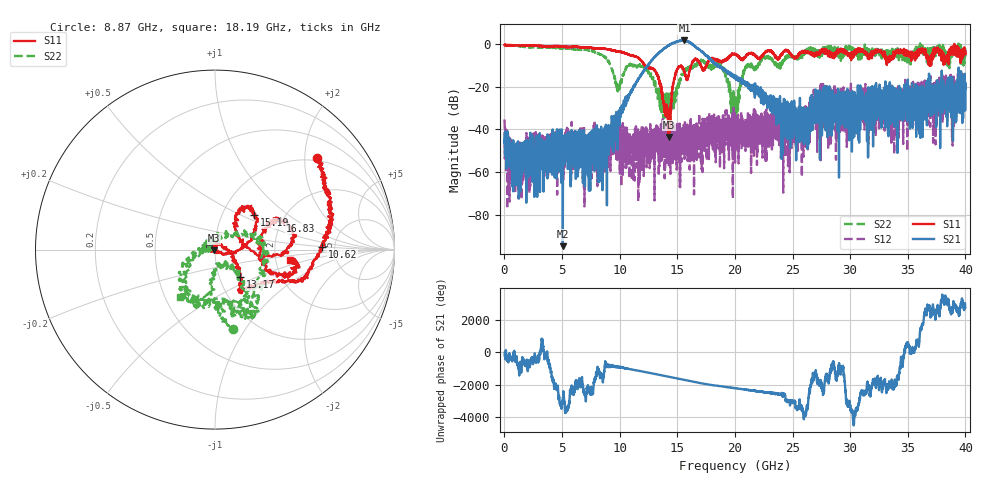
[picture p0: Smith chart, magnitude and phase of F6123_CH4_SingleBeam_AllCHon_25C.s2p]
!Keysight Technologies,N5245B,MY55451909,A.17.20.08
!Date: Tuesday, November 21, 2023 17:11:18
!Correction: S11(C  2-Port  )
!S21(C  2-Port  )
!S12(C  2-Port  )
!S22(C  2-Port  )
!S2P File: Measurements: S11, S21, S12, S22:
# Hz S  RI  R 50
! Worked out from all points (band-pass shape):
!   4000 points, 10 MHz to 40 GHz, reference 50 ohm
!   highest |S21| = 1.73 dB at 15.62 GHz (marker M1); lowest = -94.9 dB at 5.06 GHz (marker M2)
!   |S21| within 3 dB of the highest: 14.06 GHz to 16.57 GHz (2.514 GHz wide, 16.4 % of centre); 16.57504 GHz to 16.59008 GHz (15.04 MHz wide, 0.0907 % of centre)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
!   lowest |S11| = -43.5 dB at 14.26 GHz (marker M3), VSWR 1.01, Z = 49.5 - j0.431 ohm
!   |S11| at or under -10 dB: 12.21 GHz to 15.33 GHz (3.119 GHz wide, 22.7 % of centre); 15.33 GHz to 16.2 GHz (865.6 MHz wide, 5.49 % of centre); 17.04 GHz to 17.53 GHz (481.7 MHz wide, 2.79 % of centre)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
!   |S22| runs from -48.0 to 0.4 dB; largest |S21 - S12| = 1.2
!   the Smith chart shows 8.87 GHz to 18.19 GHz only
!   S11 on the Smith chart (normalised r, x): 8.87 GHz: 0.93, +2.28; 10.62 GHz: 3.94, +0.21; 13.17 GHz: 1.26, -0.40; 15.19 GHz: 1.42, +0.59; 16.83 GHz: 1.95, +0.75; 18.19 GHz: 2.40, -0.33
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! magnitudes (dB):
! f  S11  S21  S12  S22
! 10 MHz  -0.4  -42.8  -35.3  -0.8
! 260 MHz  -0.6  -45.9  -46.7  -0.8
! 1.42 GHz  -0.7  -51.6  -51.0  -1.0
! 5.06 GHz  -1.2  -94.9  -51.1  -1.9
! 6.68 GHz  -1.4  -45.4  -42.9  -2.5
! 8.87 GHz  -2.3  -42.3  -46.2  -6.9
! 9.83 GHz  -3.3  -34.5  -39.4  -22.2
! 10.62 GHz  -4.5  -26.1  -39.3  -10.9
! 13.17 GHz  -13.6  -5.4  -48.0  -21.5
! 13.34 GHz  -15.2  -4.5  -45.8  -25.2
! 14.26 GHz  -43.5  -0.6  -57.7  -23.8
! 15.19 GHz  -10.7  1.4  -44.5  -16.5
! 15.62 GHz  -12.9  1.7  -44.8  -13.1
! 16.83 GHz  -8.0  -2.3  -42.8  -8.8
! 18.19 GHz  -7.5  -8.8  -33.0  -9.7
! 19.06 GHz  -7.9  -12.0  -58.3  -11.4
! 20.01 GHz  -4.6  -15.0  -55.7  -29.9
! 21.09 GHz  -4.7  -18.8  -36.8  -10.2
! 24.22 GHz  -3.8  -33.2  -38.2  -7.5
! 26.67 GHz  -5.1  -28.5  -26.0  -2.5
! 33.34 GHz  -7.1  -31.7  -35.3  -4.0
! 40 GHz  -4.6  -21.0  -18.1  -5.7
